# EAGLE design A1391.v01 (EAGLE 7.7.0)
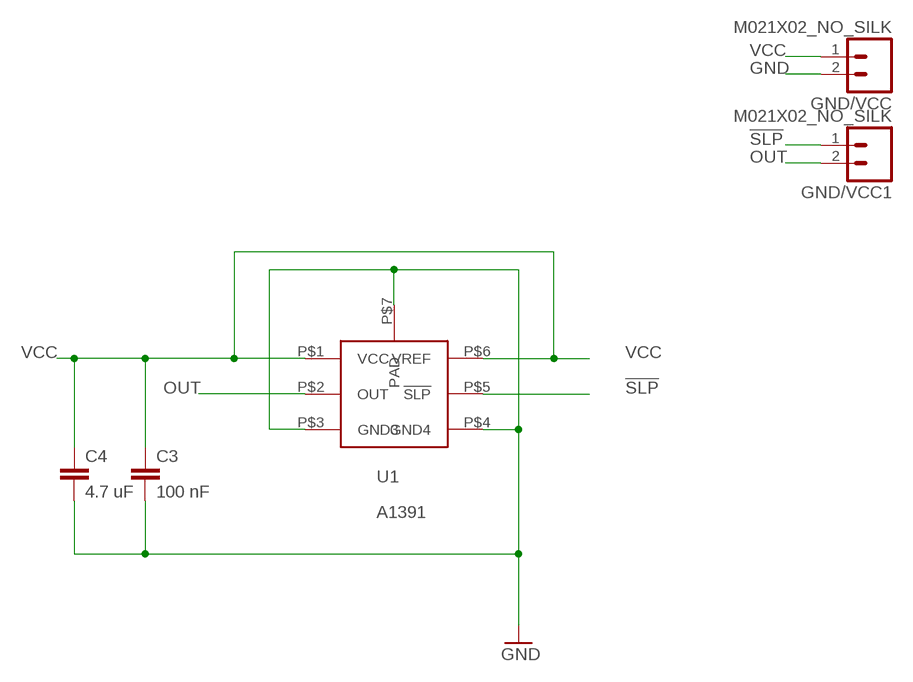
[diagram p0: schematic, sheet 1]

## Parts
C3  100 nF  0402CAP.KW  [0402-CAP]
C4  4.7 uF  0402CAP.KW  [0402-CAP]
GND/VCC  M021X02_NO_SILK  [1X02_NO_SILK]
GND/VCC1  M021X02_NO_SILK  [1X02_NO_SILK]
U1  A1391  [A1391]

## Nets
!SLP: GND/VCC1.1 U1.P$5(!SLP)
GND: C3.2 C4.2 GND/VCC.2 U1.P$3(GND3) U1.P$4(GND4) U1.P$7(PAD)
OUT: GND/VCC1.2 U1.P$2(OUT)
VCC: C3.1 C4.1 GND/VCC.1 U1.P$1(VCC) U1.P$6(VREF)

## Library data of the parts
C3 C4 = SparkFun-Capacitors:0402CAP.KW
GND/VCC GND/VCC1 = SparkFun-Connectors:M02: Standard 2-pin 0.1" header. Use with
U1 = kris:A1391: A1391 Hall Sensor

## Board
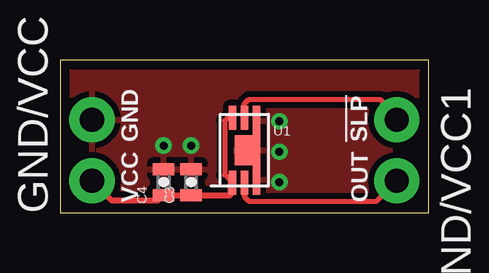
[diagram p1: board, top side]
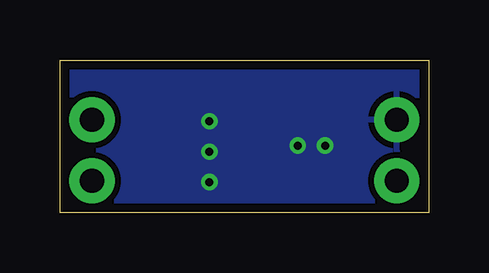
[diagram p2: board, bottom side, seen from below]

Size 15.37 x 6.36 mm. Coordinates in mm from the lower left corner, seen from the top.
Outline: 0,0 15.37,0 15.37,6.36 0,6.36 0,0
Copper layers (1*16): Top 0.0356mm / dielectric 1.5011mm / Bottom 0.0356mm
Design rules "oshpark-2layer *": minimum track width 6mil, minimum drill 13mil, track to track 6mil, track to pad 6mil, pad to pad 6mil, via to via 6mil, smd to smd 6mil, copper to edge 15mil, drill to drill 6mil, minimum pad ring 7mil, minimum via ring 7mil, stop-mask expansion 2.5mil, vias tented up to drill 20mil, thermal gap 10mil

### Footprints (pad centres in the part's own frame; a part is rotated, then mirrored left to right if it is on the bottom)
0402-CAP = smd 0.5 x 0.9: 1 -0.55,0; 2 0.55,0
1X02_NO_SILK = drill 1.016 pad 1.88: 1 0,0; 2 2.54,0
A1391 = smd 0.3 x 1: P$1 -0.5,-1.35; P$2 0,-1.35; P$5 0,1.35; P$6 -0.5,1.35 | smd 0.3 x 1.23: P$3 0.5,-1.238; P$4 0.5,1.238 | smd 1.05 x 1.25: P$7 0.125,0

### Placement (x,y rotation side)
C3  5.46,1.27 90 top
C4  4.32,1.27 90 top
GND/VCC  1.33,1.33 90 top
GND/VCC1  14.03,3.87 270 top
U1  7.68,2.6 0 top

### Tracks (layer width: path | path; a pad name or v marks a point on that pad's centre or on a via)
!SLP
  Top 0.203: U1.P$5 7.68,4.53 7.87,4.72 13.34,4.72 GND/VCC1.1
GND  (via drill 0.33)
  other vias: 4.32,2.79 5.46,2.79 9.14,3.81 9.14,1.27 9.14,2.54
  pour Bottom (isolate 0.254): 0,6.36 15.49,6.36 15.49,0 0,0
  pour Top (isolate 0.254): 0,6.36 15.49,6.36 15.49,0 0,0
OUT
  Top 0.203: U1.P$2 7.68,0.67 7.87,0.48 13.21,0.48 GND/VCC1.2
VCC
  Top 0.203: U1.P$6 6.98,3.95 6.86,3.83 6.86,1.58 U1.P$1
  Top 0.254: 7.18,1.23 U1.P$1 7.11,1.18 7.11,0.76 7.07,0.72 C3.1 C4.1 4.28,0.72 4.06,0.51 2.16,0.51 GND/VCC.1

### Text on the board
tPlace: GND | !SLP | VCC | OUT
